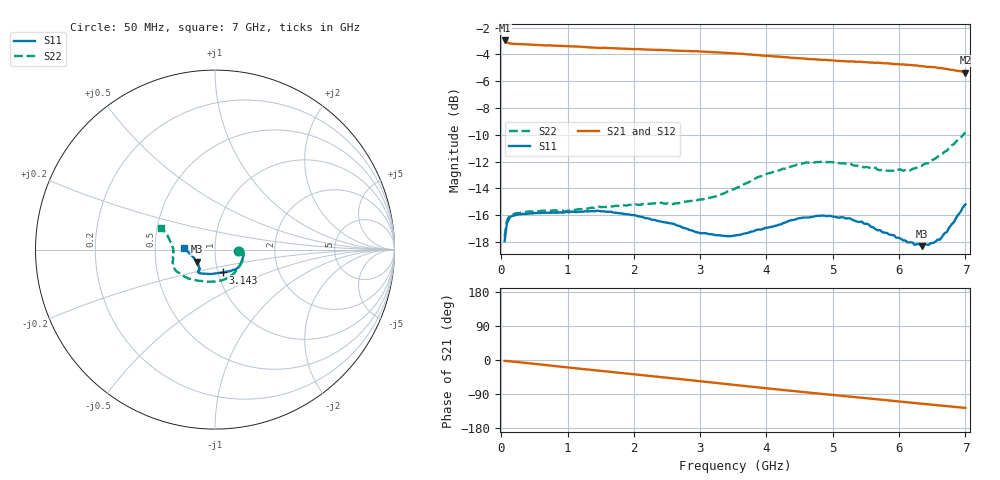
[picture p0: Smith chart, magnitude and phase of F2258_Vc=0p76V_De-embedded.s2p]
! Integrated Device Technology
! Corporate Headquarters
! 6024 Silver Creek Valley Road
! San Jose, CA 95138  USA
! Phone:  1-408-284-8200
! Toll Free:  1-800-223-1366
! Webpage:  http://www.idt.com/
! Timing and RF Division
! 515 Groton Road, Suite 102
! Westford, MA 01886-6024
! Device:  F2258
! Description: Voltage Variable RF Attenuator
! Frequency:  50.0 -  6000.00 MHz
! Package:  3x3 mm Thin QFN Plastic Package: 16 pin
! Ports:  2 RF, 2 DC
!  Pin  1  = NC
!  Pin  2  = NC
!  Pin  3  = RF2  = Port 2
!  Pin  4  = GND
!  Pin  5  = Vdd
!  Pin  6  = NC
!  Pin  7  = VCTRL
!  Pin  8  = NC
!  Pin  9  = GND
!  Pin 10  = RF1  = Port 1
!  Pin 11  = NC
!  Pin 12  = NC
!  Pin 13  = NC
!  Pin 14  = NC
!  Pin 15  = NC
!  Pin 16  = NC
! Vcntrl:  0.760 Volts
! Vdd:  +3.300 Volts
! Current:  1.128 mA
! Data:  The device was measured on a the F2258 evaluation board which has
!  individual transmission lines to the RF pins.  Data was collected
!  using a calibrated network analyzer.  The evaluation board was
!  de-embedded using a TRL calibration technique.
!  The reference plane is the edge of the package pin.
! Misc:  SN 10
!  Action Tracker AT0285
! Date Measured:  2014-12-10
! Date:  2016-01-13  MJV
! Note:
!  Integrated Device Technology supplies this data as a sample of measured
!  data at the package pin for this product.  Your particular data for this
!  product may vary.
!  Data was taken at 25 degrees C.
!  Integrated Device Technology reserves the right to change this data at anytime.
!Freq_(GHz)  S11M_(dB)  S11P_(deg)  S21M_(dB)  S21P_(deg)  S12M_(dB)  S12P_(deg)  S22M_(dB)  S22P_(deg)
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# GHz S dB R 50
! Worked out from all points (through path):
!   201 points, 50 MHz to 7 GHz, reference 50 ohm
!   highest |S21| = -2.96 dB at 50 MHz (marker M1); lowest = -5.4 dB at 7 GHz (marker M2)
!   group delay of S21, straight-line fit = 50 ps
!   lowest |S11| = -18.3 dB at 6.34 GHz (marker M3), VSWR 1.28, Z = 40.5 - j5.6 ohm
!   |S11| at or under -10 dB: start of sweep to end of sweep
!   |S22| runs from -17.6 to -9.8 dB; largest |S21 - S12| = 0.0036
!   S11 on the Smith chart (normalised r, x): 50 MHz: 1.29, -0.01; 3.143 GHz: 1.05, -0.27; 7 GHz: 0.70, +0.01
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0.05  -17.94 -2.3  -2.96 -2.2  -2.96 -2.2  -17.61 -3.1
0.08475  -16.63 -2.8  -3.10 -2.6  -3.10 -2.6  -16.42 -3.8
0.15425  -16.07 -4.1  -3.20 -3.7  -3.19 -3.7  -15.97 -6.4
0.606  -15.82 -15.8  -3.31 -12.2  -3.32 -12.2  -15.67 -22.8
0.9535  -15.78 -25.5  -3.38 -18.7  -3.37 -18.7  -15.76 -36.4
1.2315  -15.74 -31.1  -3.45 -23.9  -3.44 -23.8  -15.53 -45.7
1.6485  -15.74 -38.4  -3.54 -31.4  -3.53 -31.4  -15.35 -58.2
2.37825  -16.46 -49.9  -3.66 -44.5  -3.68 -44.5  -15.14 -78.2
2.58675  -16.63 -54.2  -3.71 -48.4  -3.74 -48.4  -15.18 -84.5
2.93425  -17.27 -64.0  -3.76 -54.8  -3.80 -54.8  -14.96 -96.8
3.14275  -17.42 -71.2  -3.83 -58.6  -3.86 -58.7  -14.71 -104.7
3.525  -17.52 -87.5  -3.94 -65.9  -3.94 -65.8  -14.03 -120.3
4.0115  -16.93 -107.8  -4.11 -74.9  -4.10 -74.9  -12.90 -137.6
4.498  -16.23 -120.8  -4.30 -83.6  -4.29 -83.6  -12.16 -150.4
4.7065  -16.12 -123.2  -4.36 -87.2  -4.35 -87.2  -12.10 -154.6
5.2625  -16.24 -127.2  -4.53 -96.7  -4.53 -96.7  -12.14 -163.8
5.85325  -17.46 -131.2  -4.68 -106.8  -4.71 -106.8  -12.68 -175.0
6.166  -18.03 -138.1  -4.79 -112.3  -4.81 -112.2  -12.67 178.0
6.33975  -18.32 -145.9  -4.88 -115.3  -4.89 -115.3  -12.33 173.3
6.61775  -17.83 -163.1  -5.03 -120.1  -5.03 -120.1  -11.56 166.1
6.722  -17.25 -169.1  -5.10 -121.9  -5.11 -121.9  -11.19 163.3
7  -15.20 177.4  -5.36 -126.4  -5.33 -126.4  -9.84 157.8
